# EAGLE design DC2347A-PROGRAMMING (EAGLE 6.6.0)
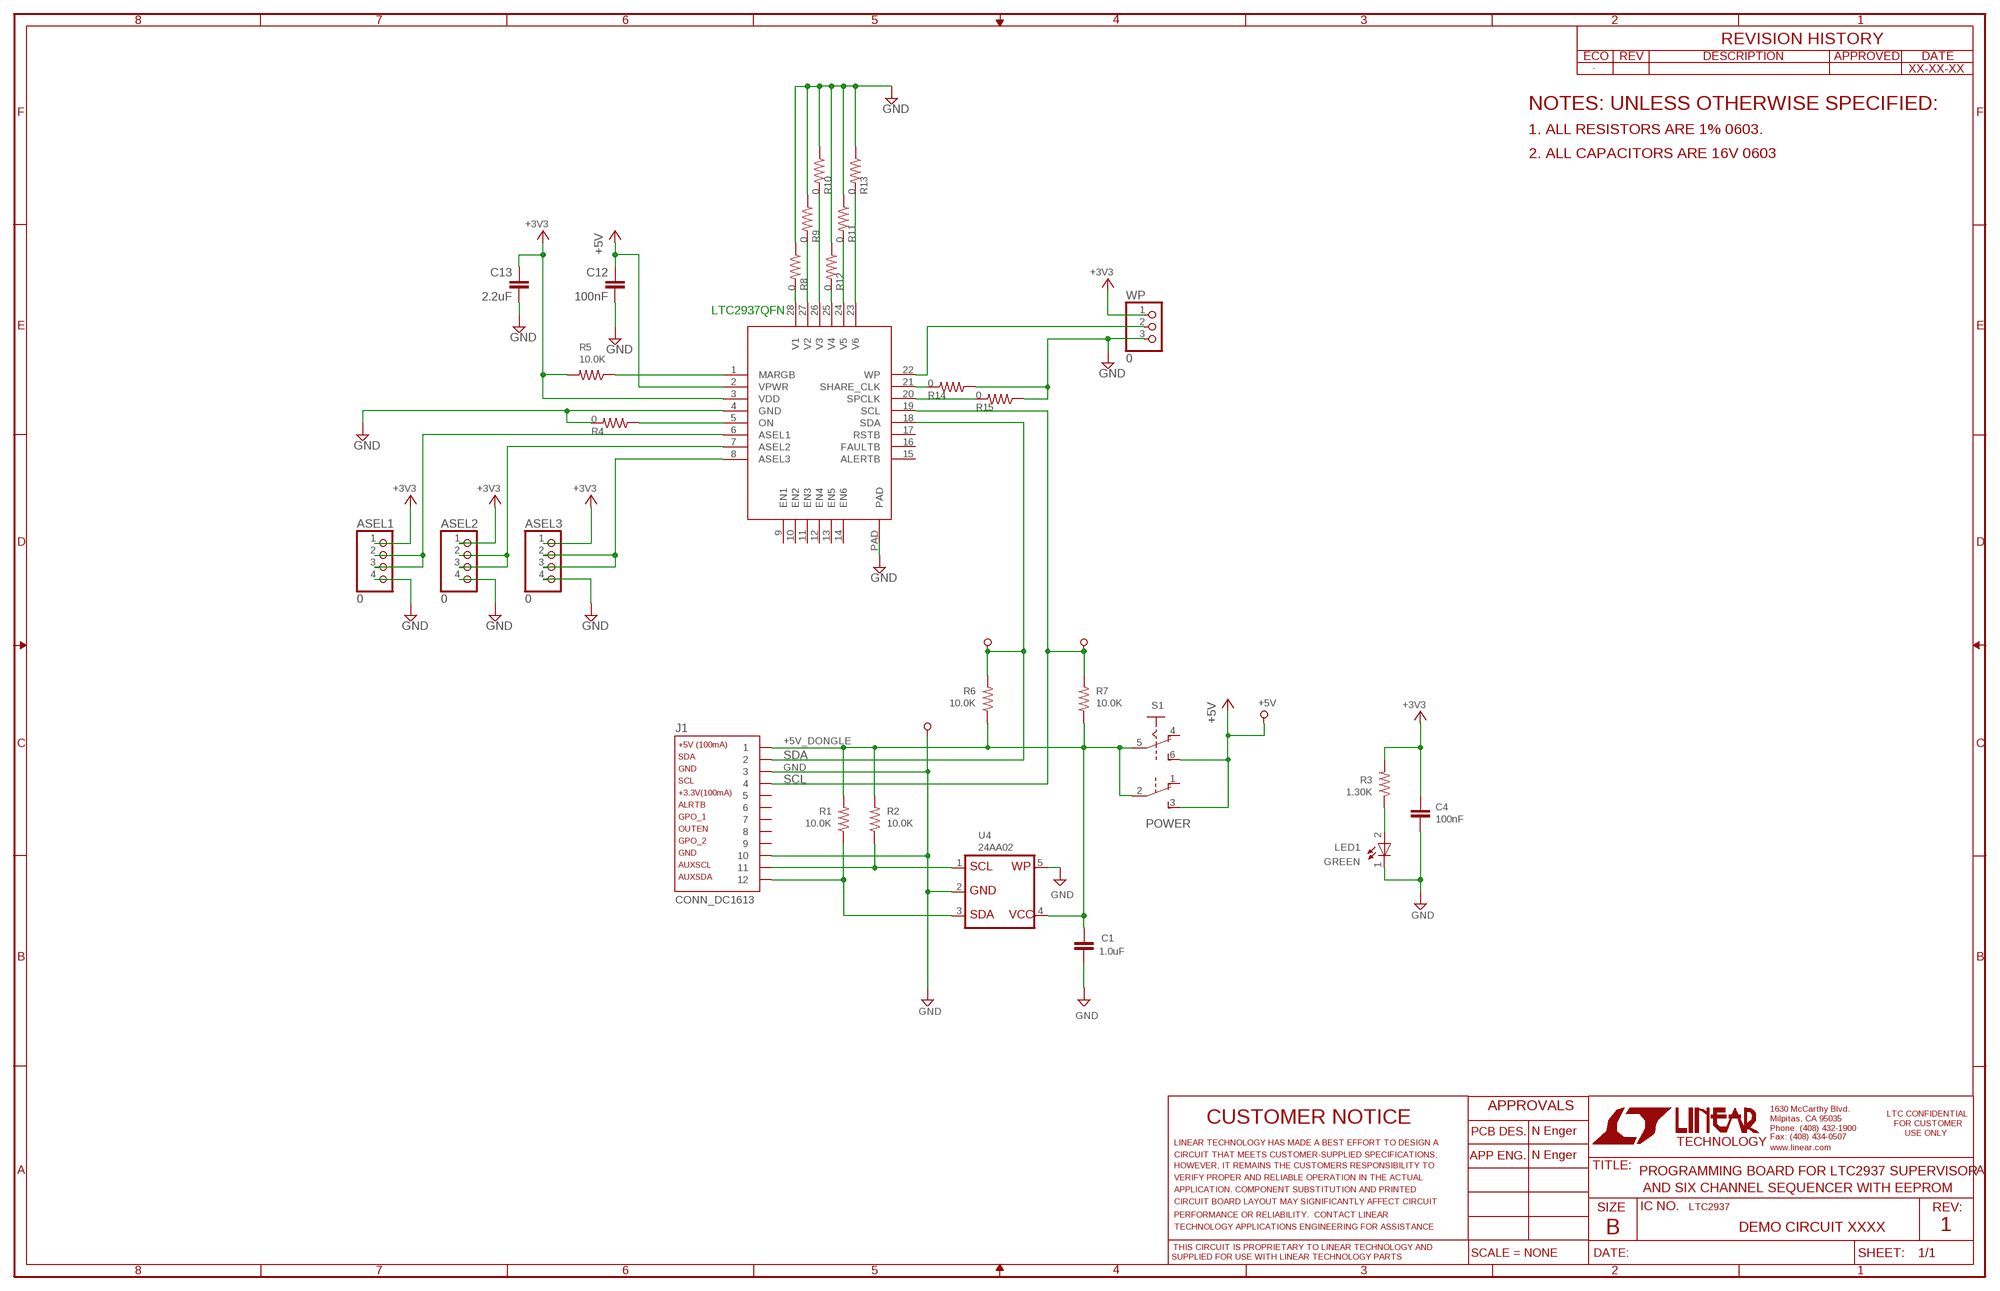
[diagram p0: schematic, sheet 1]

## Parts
ASEL1  0  PINHD-1X4  [1X04]
ASEL2  0  PINHD-1X4  [1X04]
ASEL3  0  PINHD-1X4  [1X04]
C1  1.0uF  CC0603_BOX  [C0603_BOX]
C4  100nF  CC0603_BOX  [C0603_BOX]
C12  100nF  CC0603_BOX  [C0603_BOX]
C13  2.2uF  CC0603_BOX  [C0603_BOX]
J1  CONN_DC1613  [CONN_DC1613]
LED1  LED-0603  [CHIPLED_0603]
R1  10.0K  RR0603_BOX  [R0603_BOX]
R2  10.0K  RR0603_BOX  [R0603_BOX]
R3  1.30K  RR0603_BOX  [R0603_BOX]
R4  0  RR0603_BOX  [R0603_BOX]
R5  10.0K  RR0603_BOX  [R0603_BOX]
R6  10.0K  RR0603_BOX  [R0603_BOX]
R7  10.0K  RR0603_BOX  [R0603_BOX]
R8  0  RR0603_BOX  [R0603_BOX]
R9  0  RR0603_BOX  [R0603_BOX]
R10  0  RR0603_BOX  [R0603_BOX]
R11  0  RR0603_BOX  [R0603_BOX]
R12  0  RR0603_BOX  [R0603_BOX]
R13  0  RR0603_BOX  [R0603_BOX]
R14  0  RR0603_BOX  [R0603_BOX]
R15  0  RR0603_BOX  [R0603_BOX]
S1  POWER  JS202011CQN  [JS202011CQN]
TP1  TESTPOINT_BIG  [TP1]
TP2  TESTPOINT_BIG  [TP1]
TP3  TESTPOINT_BIG  [TP1]
TP4  TESTPOINT_BIG  [TP1]
U4  24AA02  [SOT-23-5]
U$1  LTC2937-SOCKET  [SOCKET-QFN-28-6X5]
WP  0  PINHD-1X3  [1X03]

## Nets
+3V3: ASEL1.1 ASEL2.1 ASEL3.1 C4.1 C13.1 R3.2 R5.2 U$1.3(VDD) WP.1
+5V: C12.1 S1.3(B:S) S1.6(A:S) TP1.TP U$1.2(VPWR)
+5V_DONGLE: C1.1 J1.1 R1.2 R2.2 R6.1 R7.1 S1.2(B:P) S1.5(A:P) U4.4
GND: ASEL1.4 ASEL2.4 ASEL3.4 C1.2 C4.2 C12.2 C13.2 J1.3 J1.10 LED1.C R4.2 R8.1 R9.1 R10.1 R11.1 R12.1 R13.1 R14.1 R15.1 TP4.TP U4.2 U4.5 U$1.4(GND) U$1.PAD WP.3
N$1: R8.2 U$1.28(V1)
N$2: R5.1 U$1.1(MARGB)
N$3: R9.2 U$1.27(V2)
N$4: ASEL1.2 ASEL1.3 U$1.6(ASEL1)
N$5: J1.11 R2.1 U4.1
N$6: J1.12 R1.1 U4.3
N$7: R4.1 U$1.5(ON)
N$8: R10.2 U$1.26(V3)
N$9: LED1.A R3.1
N$10: R11.2 U$1.24(V5)
N$11: ASEL2.2 ASEL2.3 U$1.7(ASEL2)
N$12: R12.2 U$1.25(V4)
N$13: R13.2 U$1.23(V6)
N$14: U$1.22(WP) WP.2
N$15: R14.2 U$1.21(SHARE_CLK)
N$16: ASEL3.2 ASEL3.3 U$1.8(ASEL3)
N$17: R15.2 U$1.20(SPCLK)
SCL: J1.4 R7.2 TP2.TP U$1.19(SCL)
SDA: J1.2 R6.2 TP3.TP U$1.18(SDA)
Unconnected: J1.5 J1.6 J1.7 J1.8 J1.9 S1.1(B:O) S1.4(A:O) U$1.9(EN1) U$1.10(EN2) U$1.11(EN3) U$1.12(EN4) U$1.13(EN5) U$1.14(EN6) U$1.15(ALERTB) U$1.16(FAULTB) U$1.17(RSTB)

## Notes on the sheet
- XX-XX-XX
- NOTES: UNLESS OTHERWISE SPECIFIED:
- 1. ALL RESISTORS ARE 1% 0603.
- 2. ALL CAPACITORS ARE 16V 0603
- LTC2937QFN
- GREEN
- N Enger
- N Enger
- PROGRAMMING BOARD FOR LTC2937 SUPERVISOR
- AND SIX CHANNEL SEQUENCER WITH EEPROM
- LTC2937
- DEMO CIRCUIT XXXX | 1

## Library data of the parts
ASEL1-ASEL3 = pinhead:PINHD-1X4: PIN HEADER
C1 C4 C12 C13 = kalin:C: CAPACITOR, European symbol
J1 = kalin:CONN_DC1613: Connector for LT DC1613 USB Dongle
LED1 = kalin:LED-0603: SMD LED in R0603
R1-R15 = kalin:R: RESISTOR, American symbol
S1 = nengerLib:JS202011CQN: SLIDING SWITCH Siemens, distributor Buerklin, 11G766
TP1-TP4 = kalin:TESTPOINT_BIG: Large Test Point
U4 = kalin:24AA02: 2Kbit I2C Serial EEPROM
U$1 = nengerLib:LTC2937-SOCKET: ltc2937 Socket
WP = pinhead:PINHD-1X3: PIN HEADER

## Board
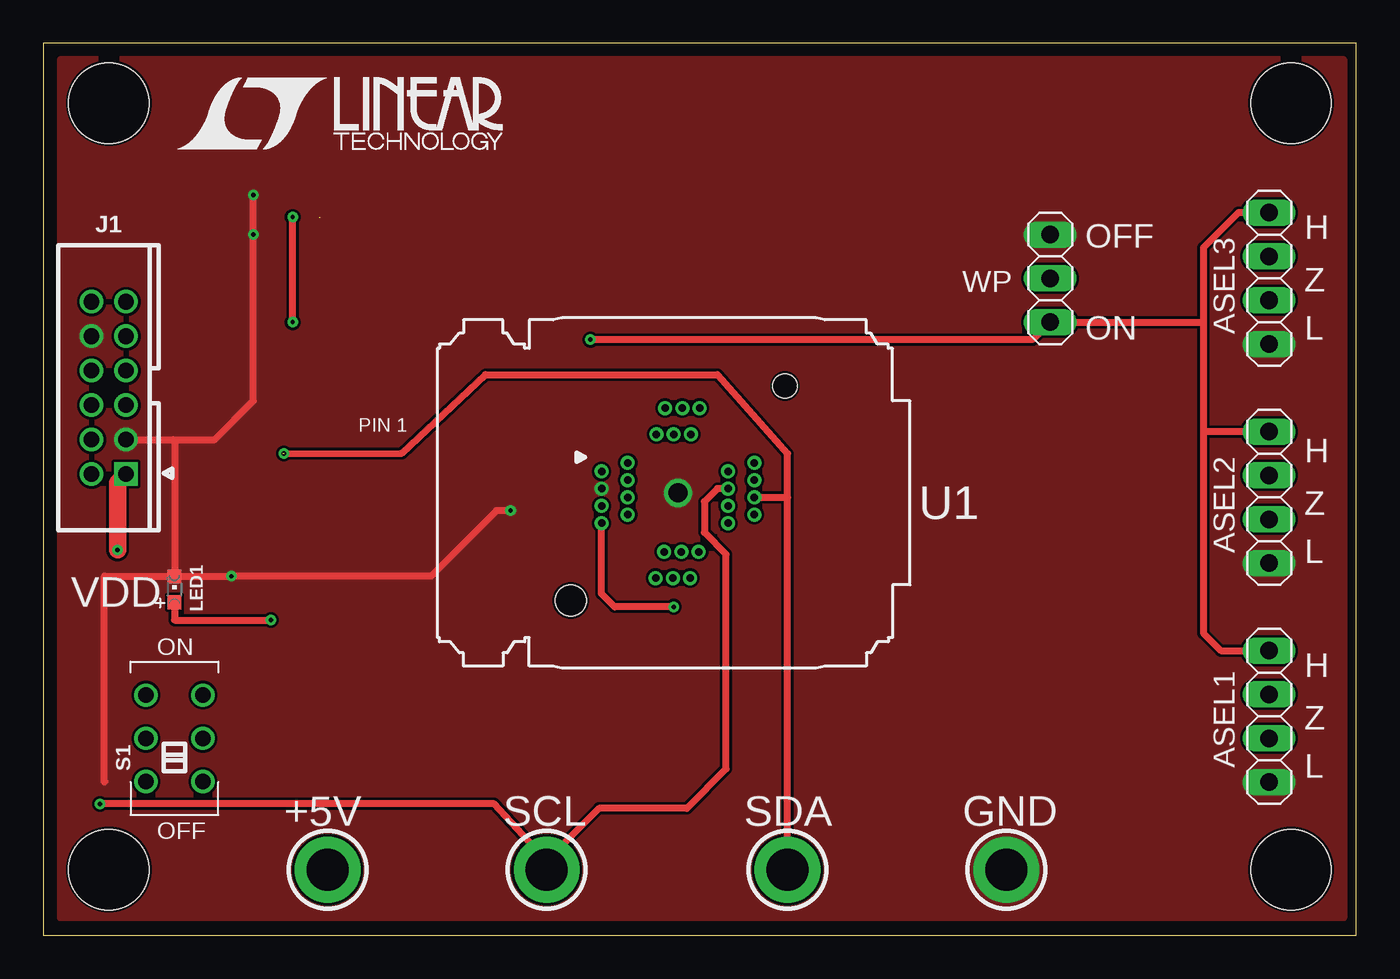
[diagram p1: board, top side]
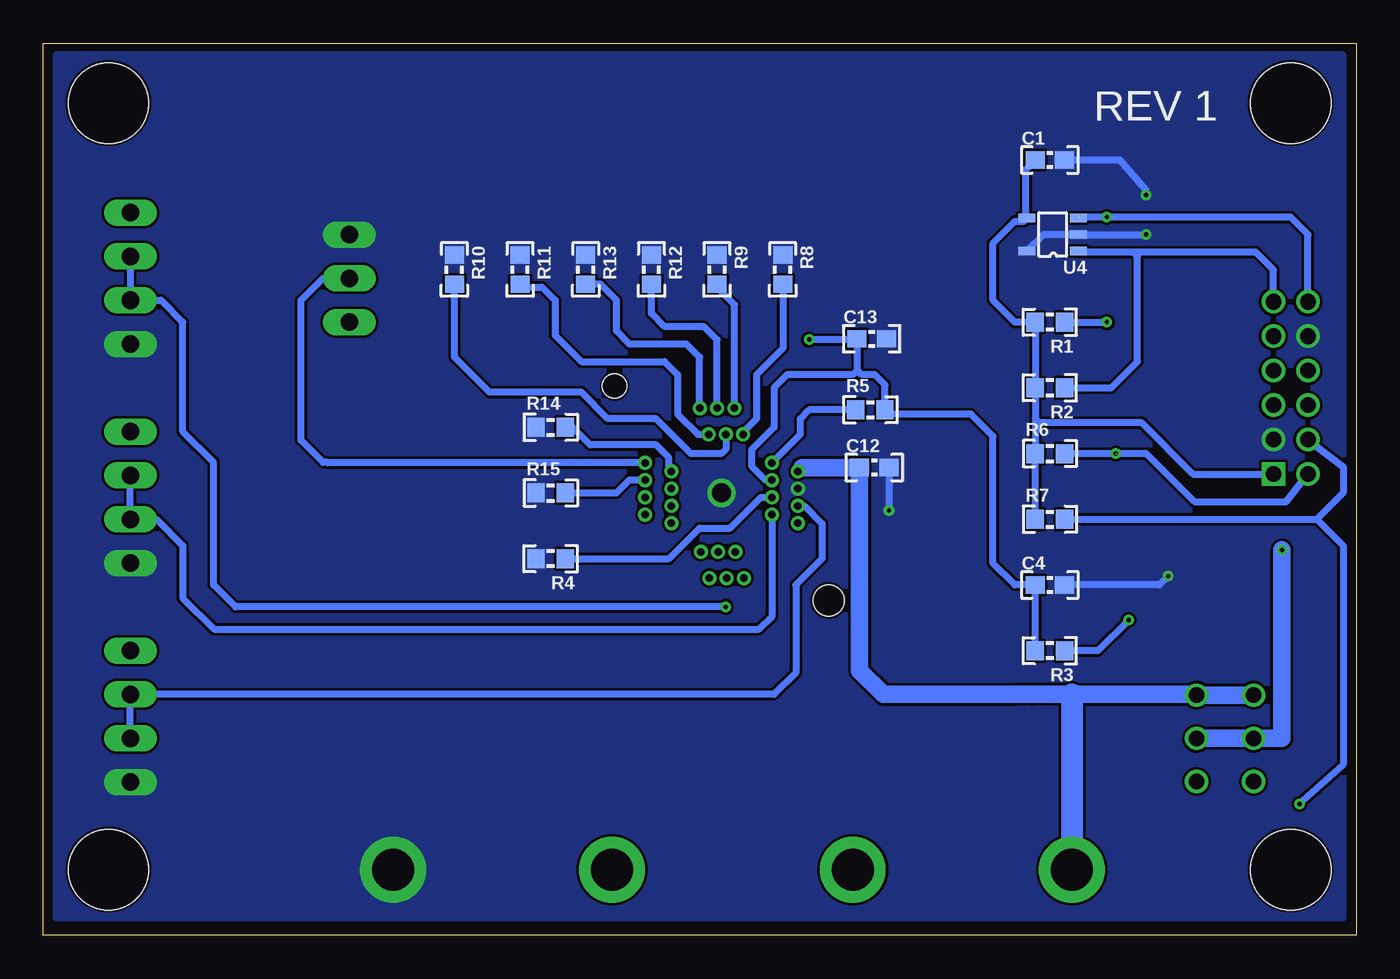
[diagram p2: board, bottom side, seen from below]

Size 76.18 x 51.74 mm. Coordinates in mm from the lower left corner, seen from the top.
Outline: 0,0 76.18,0 76.18,51.74 0,51.74 0,0
Copper layers (1*2+15*16): Top 0.071mm / dielectric 0.114mm / Route2 0.036mm / dielectric 39mil / Route15 0.036mm / dielectric 0.114mm / Bottom 0.071mm
Design rules "nenger *": minimum track width 6mil, minimum drill 8mil, track to track 6mil, track to pad 6mil, pad to pad 6mil, via to via 6mil, smd to smd 6mil, copper to edge 6mil, drill to drill 8mil, minimum pad ring 7mil, minimum via ring 7mil, stop-mask expansion 3mil, vias tented up to drill 3mil, thermal gap 10mil
Holes 4.65 mm at 3.81,48.26 3.81,3.81 72.39,3.81 72.39,48.26

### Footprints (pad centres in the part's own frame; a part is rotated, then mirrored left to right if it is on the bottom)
1X04 = drill 1.016 long: 1 -3.81,0; 2 -1.27,0; 3 1.27,0; 4 3.81,0
C0603_BOX = smd 1.1 x 1: 1 -0.85,0; 2 0.85,0
CONN_DC1613 = drill 0.914 square: 1 -5,-1 | drill 0.914: 2 -5,1; 3 -3,-1; 4 -3,1; 5 -1,-1; 6 -1,1; 7 1,-1; 8 1,1; 9 3,-1; 10 3,1; 11 5,-1; 12 5,1
CHIPLED_0603 = smd 0.8 x 0.8: A 0,-0.75; C 0,0.75
R0603_BOX = smd 1 x 1.1: 1 -0.85,0; 2 0.85,0
JS202011CQN = drill 0.9: 1 -2.5,1.65; 2 0,1.65; 3 2.5,1.65; 4 -2.5,-1.65; 5 0,-1.65; 6 2.5,-1.65
TP1 = drill 2.438 pad 3.81: TP 0,0
SOT-23-5 = smd 1 x 0.5: 1 -1.649,0.95; 2 -1.649,0; 3 -1.649,-0.95; 4 1.333,-0.95; 5 1.333,0.95
SOCKET-QFN-28-6X5 = drill 0.432 pad 0.813: 1 -2.92,1.75; 2 -4.435,1.25; 3 -2.92,0.75; 4 -4.435,0.25; 5 -2.92,-0.25; 6 -4.435,-0.75; 7 -2.92,-1.25; 8 -4.435,-1.75; 9 -1.3,-4.935; 10 -0.8,-3.41; 11 -0.3,-4.935; 12 0.2,-3.41; 13 0.7,-4.935; 14 1.2,-3.41; 15 2.9,-1.75; 16 4.425,-1.25; 17 2.9,-0.75; 18 4.425,-0.25; 19 2.9,0.25; 20 4.425,0.75; 21 2.9,1.25; 22 4.425,1.75; 23 1.25,4.925; 24 0.75,3.4; 25 0.25,4.925; 26 -0.25,3.4; 27 -0.75,4.925; 28 -1.25,3.4 | drill 1.1: PAD 0,0 | hole 1.803: -6.223,-6.233 | hole 1.397: 6.203,6.203
1X03 = drill 1.016 long: 1 -2.54,0; 2 0,0; 3 2.54,0

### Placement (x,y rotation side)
ASEL1  71.12,12.7 270 top
ASEL2  71.12,25.4 270 top
ASEL3  71.12,38.1 270 top
C1  17.78,44.96 0 bottom
C4  17.78,20.32 0 bottom
C12  27.97,27.13 0 bottom
C13  28.12,34.59 0 bottom
J1  3.81,31.75 90 top
LED1  7.62,20.07 0 top
R1  17.78,35.56 180 bottom
R2  17.78,31.75 180 bottom
R3  17.78,16.51 180 bottom
R4  46.74,21.84 180 bottom
R5  28.19,30.48 0 bottom
R6  17.78,27.94 0 bottom
R7  17.78,24.13 0 bottom
R8  33.27,38.61 270 bottom
R9  37.08,38.61 270 bottom
R10  52.32,38.61 270 bottom
R11  48.51,38.61 270 bottom
R12  40.89,38.61 270 bottom
R13  44.7,38.61 270 bottom
R14  46.74,29.46 0 bottom
R15  46.74,25.65 0 bottom
S1  7.62,11.43 90 top
TP1  16.51,3.81 0 top
TP2  29.21,3.81 0 top
TP3  43.18,3.81 0 top
TP4  55.88,3.81 0 top
U4  17.78,40.64 180 bottom
U$1  36.83,25.65 0 top
U$3  [LT_LOGO_LARGE]  7.62,45.47 0 top
WP  58.42,38.1 90 top

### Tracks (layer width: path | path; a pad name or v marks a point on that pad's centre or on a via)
+3V3  (via drill 0.25)
  Top 0.406: ASEL3.1 69.34,41.91 67.31,39.88 67.31,35.5 | 67.31,35.5 67.31,29.21 | 67.31,29.21 67.31,17.53 68.33,16.51 ASEL1.1 | ASEL2.1 67.31,29.21 | 67.31,35.5 67.25,35.56 WP.1 57.4,34.54 v31.75,34.54
  Bottom 0.406: R3.2 C4.1 19.81,20.32 21.08,21.59 21.08,28.96 22.35,30.23 27.09,30.23 R5.2 27.34,31.92 27.94,32.51 28.7,32.51 28.96,32.77 | U$1.3 34.28,26.4 35.05,27.18 35.05,28.19 33.78,29.46 33.78,31.75 33.02,32.51 29.21,32.51 28.96,32.77 | 28.96,32.77 28.96,34.58 C13.1 29.02,34.54 v31.75,34.54
+5V
  Bottom 0.406: 11.72,13.93 S1.6 9.31,13.97 | 32.17,27.13 U$1.2
  Bottom 1.016: S1.3 S1.6 | 9.31,13.97 16.51,13.97 18.8,13.97 19.81,13.97 27.43,13.97 28.82,15.35 C12.1 32.17,27.13
  Bottom 1.27: 16.51,13.97 TP1.TP
+5V_DONGLE  (via drill 0.25)
  Top 1.016: v4.32,22.35 4.32,26.26 J1.1
  Bottom 0.406: 18.63,29.97 R2.2 R1.2 19.81,35.56 21.08,36.83 21.08,40.13 19.81,41.4 19.3,41.4 U4.4 19.18,41.66 19.18,44.41 C1.1 | 18.63,29.97 R6.1 R7.1 | J1.1 4.91,26.75 | 18.63,29.97 18.38,29.72 12.45,29.72 9.48,26.75 4.91,26.75 | 4.91,26.75 4.83,26.67
  Bottom 1.016: S1.5 S1.2 4.32,11.43 v4.32,22.35
GND  (via drill 0.25)
  Top 0.406: v12.19,42.93 v12.19,40.64 12.19,30.99 9.95,28.75 7.57,28.75 | J1.3 7.57,28.75 | 7.57,28.75 7.62,28.7 LED1.C | 3.6,8.93 3.56,8.89 3.56,20.83 7.61,20.83 LED1.C | v27.12,24.63 26.29,24.63 22.52,20.83 v10.92,20.83 10.92,20.82 LED1.C
  Bottom 0.406: v12.19,40.64 U4.2 18.16,40.64 U4.5 | v10.92,20.83 11.43,20.32 C4.2 | C12.2 v27.12,24.63 | v12.19,42.93 12.19,43.18 13.72,44.96 C1.2
  pour Top (no thermals): 1.02,50.8 75.18,50.8 75.44,50.8 75.44,1.02 1.02,1.02
  pour Bottom (no thermals): 0.76,51.05 75.44,51.05 75.44,40.89 75.44,1.02 1.02,1.02 0.76,1.02
N$1
  Bottom 0.406: R8.2 33.27,34.04 34.8,32.51 34.8,29.97 35.58,29.19 U$1.28
N$2
  Bottom 0.406: R5.1 29.07,30.5 29.09,30.48 31.75,30.48 32.26,29.97 32.26,29.06 U$1.1
N$3
  Bottom 0.406: U$1.27 36.07,30.59 36.07,36.58 37.08,37.59 R9.2
N$4
  Bottom 0.406: ASEL1.3 ASEL1.2 33.78,13.97 32.51,15.24 32.51,20.32 30.99,21.84 30.99,23.88 32.02,24.9 U$1.6
N$5
  Bottom 0.406: 4.81,36.83 J1.11 4.81,38.59 5.84,39.62 12.95,39.62 | U4.1 16.07,39.62 12.95,39.62 | R2.1 14.22,31.75 12.7,33.27 12.7,39.37 12.95,39.62
N$6  (via drill 0.25)  (1 unrouted)
  Top 0.406: v14.48,35.56 v14.48,41.66
  Bottom 0.406: 16,41.66 3.81,41.66 2.79,40.64 2.81,40.62 J1.12 | R1.1 v14.48,35.56 | v14.48,41.66 16.07,41.66 U4.3
N$7
  Bottom 0.406: R4.1 39.88,21.84 38.1,23.62 36.32,23.62 34.54,25.4 U$1.5
N$8
  Bottom 0.406: U$1.26 36.58,28.19 36.83,27.94 38.61,27.94 40.64,29.97 43.43,29.97 44.96,31.5 50.29,31.5 52.32,33.53 R10.2
N$9  (via drill 0.25)
  Top 0.406: 13.2,18.3 v13.21,18.29 7.63,18.29 LED1.A
  Bottom 0.406: v13.21,18.29 14.99,16.51 R3.1
N$10
  Bottom 0.406: R11.2 48.35,37.59 47.24,37.59 46.48,36.83 46.48,34.8 44.96,33.27 40.13,33.27 39.37,32.51 39.37,30.23 38.2,29.05 U$1.24
N$11
  Bottom 0.406: ASEL2.2 ASEL2.3 69.6,24.13 68.07,22.61 68.07,19.56 66.27,17.75 34.65,17.75 33.91,18.49 U$1.7
N$12
  Bottom 0.406: U$1.25 37.08,34.54 37.85,35.31 40.13,35.31 40.89,36.07 R12.2
N$13
  Bottom 0.406: U$1.23 38.1,30.6 38.1,33.53 38.86,34.29 42.16,34.29 42.93,35.05 42.93,36.83 43.85,37.76 R13.2
N$14
  Bottom 0.406: U$1.22 59.66,27.4 59.69,27.43 59.94,27.43 61.21,28.7 61.21,36.83 59.94,38.1 WP.2
N$15
  Bottom 0.406: U$1.21 39.88,27.05 39.88,27.69 40.64,28.45 44.45,28.45 45.47,29.46 R14.2
N$16  (via drill 0.25)
  Top 0.406: v36.58,19.05 33.15,19.05 32.38,19.81 U$1.8
  Bottom 0.406: v36.58,19.05 65.02,19.05 66.29,20.32 66.29,27.43 68.07,29.21 68.07,35.56 69.34,36.83 ASEL3.3 ASEL3.2
N$17
  Bottom 0.406: R15.2 42.93,25.65 42.16,26.42 41.27,26.42 U$1.20
SCL  (via drill 0.25)
  Top 0.406: TP2.TP 29.21,4.32 | 29.21,4.32 26.16,7.62 v3.3,7.62 | U$1.19 39.11,25.9 38.35,25.15 38.35,23.37 39.62,22.1 39.62,9.65 37.34,7.37 32.26,7.37 29.21,4.32
  Bottom 0.406: J1.4 0.76,27.18 0.76,25.65 2.29,24.13 | 2.29,24.13 0.76,22.61 0.76,9.91 v3.3,7.62 | R7.2 2.29,24.13
SDA  (via drill 0.25)  (1 unrouted)
  Top 0.406: TP3.TP 43.18,25.4 | 43.18,25.4 43.18,27.94 39.12,32.51 25.65,32.51 20.82,27.96 13.88,27.94 | U$1.18 43.18,25.4
  Bottom 0.406: R6.2 v13.97,27.94 12.19,27.94 9.4,25.15 4.06,25.15 J1.2

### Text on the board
tPlace: ON | OFF
tNames: OFF | H | Z | ON | L | PIN 1 | H | U1 | Z | L | VDD | H | Z | L | +5V | SCL | SDA | GND
bNames: REV 1
tStop: DEMO CIRCUIT 2347A | WWW.LINEAR.COM | PROGRAMMING BOARD FOR LTC2937 | (408) 432-1900
bStop: LTC CONFIDENTIAL / FOR CUSTOMER USE ONLY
